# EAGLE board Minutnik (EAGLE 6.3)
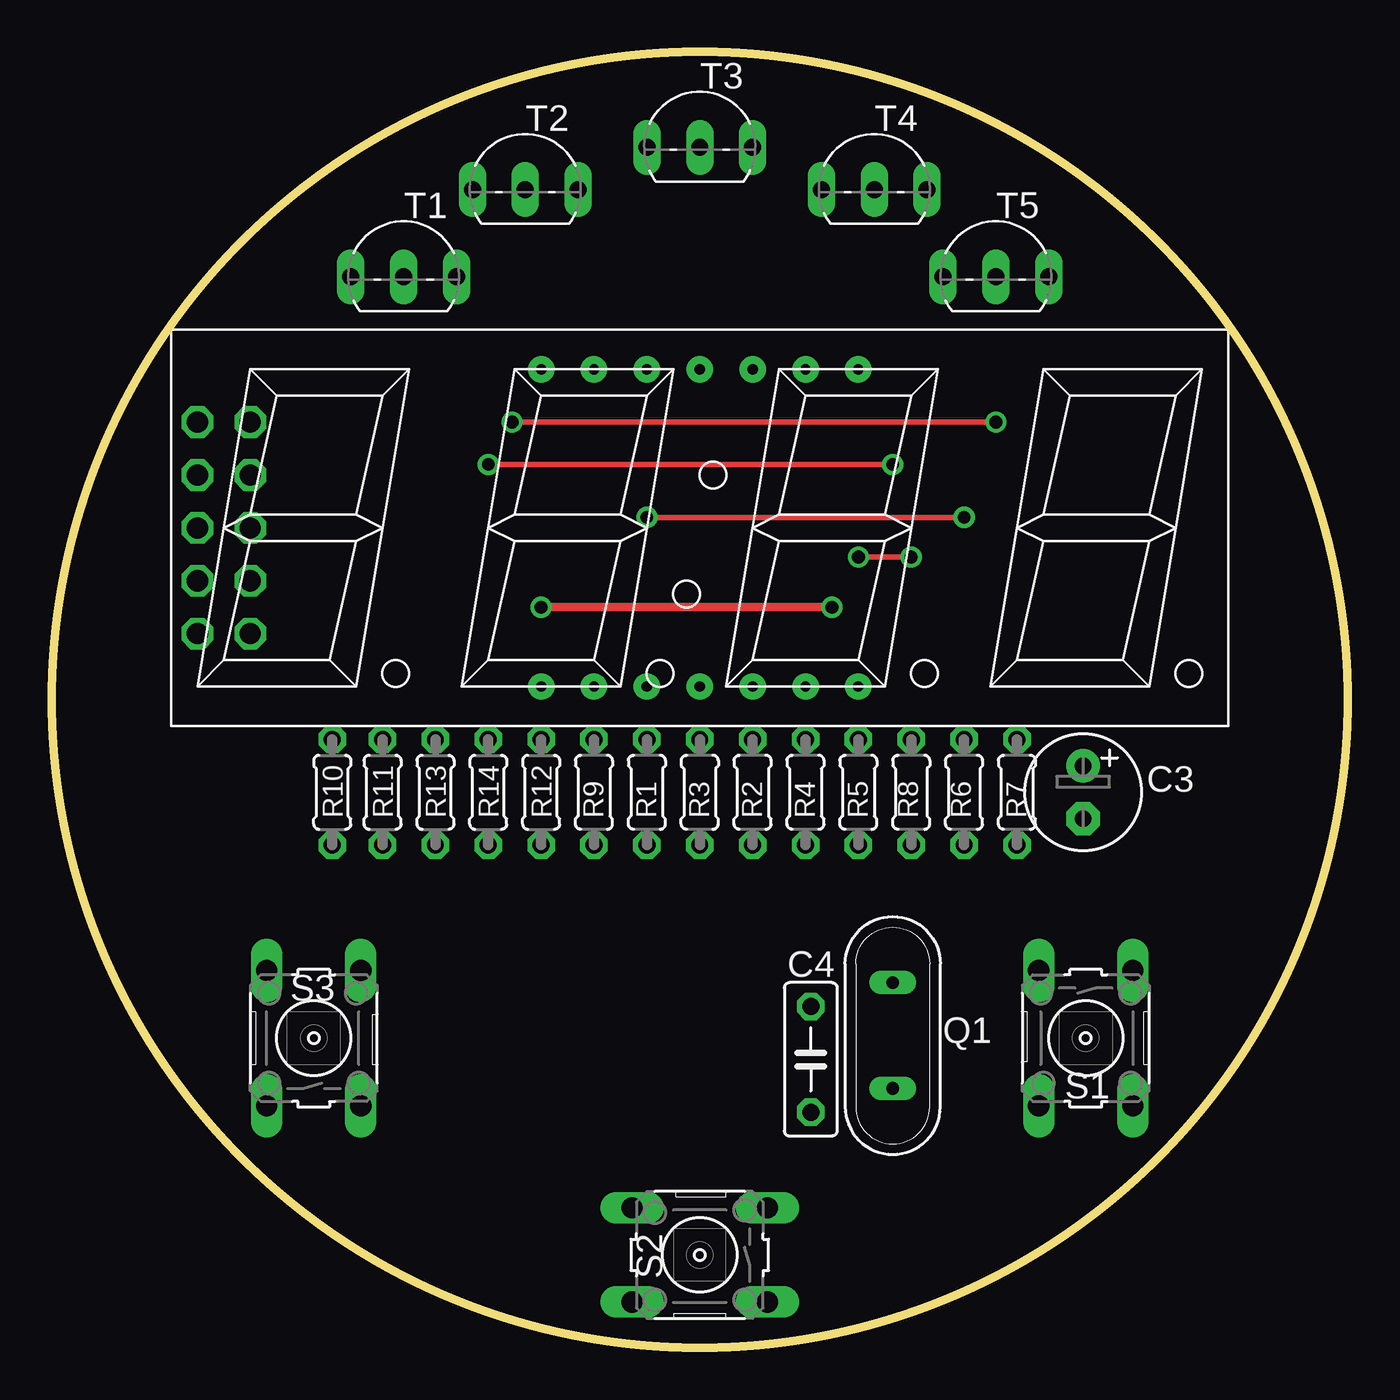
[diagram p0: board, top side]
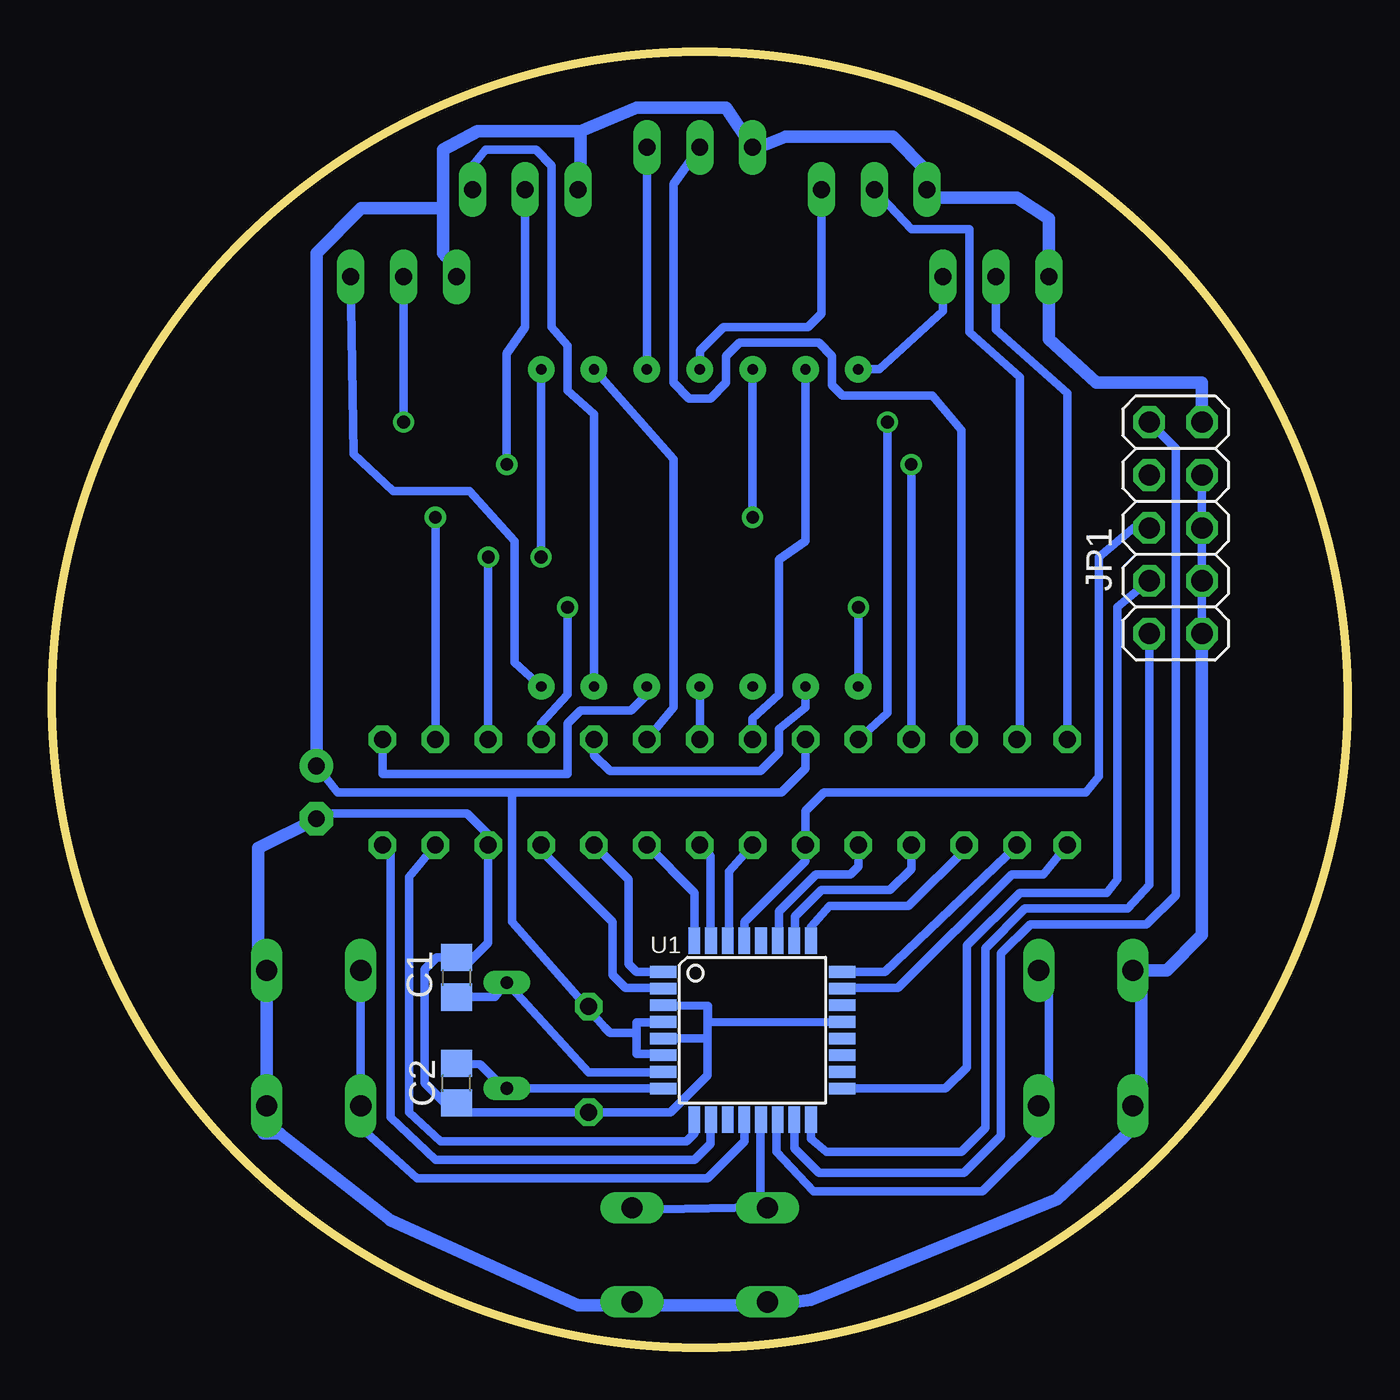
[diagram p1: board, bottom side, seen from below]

Size 62.23 x 62.23 mm. Coordinates in mm from the lower left corner, seen from the top.
Outline: circle at 31.11,31.11 radius 31.11
Copper layers (1*16): Top 0.035mm / dielectric 1.5mm / Bottom 0.035mm
Design rules "default": minimum track width 10mil, minimum drill 24mil, track to track 8mil, track to pad 8mil, pad to pad 8mil, via to via 8mil, smd to smd 8mil, copper to edge 40mil, drill to drill 8mil, minimum pad ring 10mil, minimum via ring 8mil, stop-mask expansion 4mil, vias tented up to drill 0mil, thermal gap 10mil

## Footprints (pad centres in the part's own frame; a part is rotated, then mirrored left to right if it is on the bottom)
C0805 = smd 1.3 x 1.5: 1 -0.95,0; 2 0.95,0
E2,5-6 = drill 0.813 pad 1.6: + -1.27,0 | drill 0.813 pad 1.6 octagon: - 1.27,0
C050-025X075 = drill 0.813 octagon: 1 -2.54,0; 2 2.54,0
2X05 = drill 1.016 octagon: 1 -5.08,-1.27; 2 -5.08,1.27; 3 -2.54,-1.27; 4 -2.54,1.27; 5 0,-1.27; 6 0,1.27; 7 2.54,-1.27; 8 2.54,1.27; 9 5.08,-1.27; 10 5.08,1.27
QS = drill 0.61 long: 1 -2.54,0; 2 2.54,0
0204/5 = drill 0.813 octagon: 1 -2.54,0; 2 2.54,0
B3F-10XX = drill 1.016 long: 1 -3.251,2.261; 2 3.251,2.261; 3 -3.251,-2.261; 4 3.251,-2.261
TO92-EBC = drill 0.813 long: B 0,-1.27; C -2.54,-1.27; E 2.54,-1.27
TQFP32-08 = smd 1.27 x 0.559: 1 -4.293,2.8; 2 -4.293,2; 3 -4.293,1.2; 4 -4.293,0.4; 5 -4.293,-0.4; 6 -4.293,-1.2; 7 -4.293,-2; 8 -4.293,-2.8; 17 4.293,-2.8; 18 4.293,-2; 19 4.293,-1.2; 20 4.293,-0.4; 21 4.293,0.4; 22 4.293,1.2; 23 4.293,2; 24 4.293,2.8 | smd 0.559 x 1.27: 9 -2.8,-4.293; 10 -2,-4.293; 11 -1.2,-4.293; 12 -0.4,-4.293; 13 0.4,-4.293; 14 1.2,-4.293; 15 2,-4.293; 16 2.8,-4.293; 25 2.8,4.293; 26 2,4.293; 27 1.2,4.293; 28 0.4,4.293; 29 -0.4,4.293; 30 -1.2,4.293; 31 -2,4.293; 32 -2.8,4.293
TOF-5462DX = drill 0.5 pad 1.27: A -5.08,7.62; A1 -7.62,7.62; A2 0,7.62; A3 2.54,7.62; A4 5.08,-7.62; ADOT 7.62,-7.62; B 5.08,7.62; C 0,-7.62; D -5.08,-7.62; DOT 7.62,7.62; DP -2.54,-7.62; E -7.62,-7.62; F -2.54,7.62; G 2.54,-7.62

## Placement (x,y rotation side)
C1  22pF  [C0805]  42.8,17.78 270 bottom
C2  22pF  [C0805]  42.8,12.7 90 bottom
C3  100uF  [E2,5-6]  49.53,26.67 270 top
C4  100nF  [C050-025X075]  36.45,13.84 270 top
JP1  [2X05]  8.25,39.37 270 bottom
Q1  [QS]  40.39,14.99 90 top
R1  [0204/5]  28.57,26.67 90 top
R2  [0204/5]  33.66,26.67 90 top
R3  [0204/5]  31.11,26.67 90 top
R4  [0204/5]  36.19,26.67 90 top
R5  [0204/5]  38.73,26.67 90 top
R6  [0204/5]  43.81,26.67 90 top
R7  [0204/5]  46.36,26.67 90 top
R8  [0204/5]  41.27,26.67 90 top
R9  1k  [0204/5]  26.04,26.67 90 top
R10  10k  [0204/5]  13.46,26.67 270 top
R11  10k  [0204/5]  15.88,26.67 270 top
R12  10k  [0204/5]  23.49,26.67 270 top
R13  10k  [0204/5]  18.41,26.67 270 top
R14  10k  [0204/5]  20.95,26.67 270 top
S1  [B3F-10XX]  49.66,14.86 270 top
S2  [B3F-10XX]  31.11,4.44 180 top
S3  [B3F-10XX]  12.57,14.86 90 top
T1  BC548  [TO92-EBC]  16.89,52.7 0 top
T2  BC548  [TO92-EBC]  22.73,56.9 0 top
T3  BC548  [TO92-EBC]  31.11,58.93 0 top
T4  BC548  [TO92-EBC]  39.5,56.9 0 top
T5  BC548  [TO92-EBC]  45.34,52.7 0 top
U1  ATmega8L  [TQFP32-08]  28.57,15.24 0 bottom
U$1  TOF-5462DX  [TOF-5462DX]  31.11,39.37 0 top

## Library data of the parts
C1-C4 R1-R14 = rcl
JP1 = pinhead
Q1 = special
S1-S3 = switch-omron
T1-T5 = transistor-npn
U1 = atmel
U$1 = 7seg led disp

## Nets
+5V: C3.+ C4.1 JP1.2 R9.2 T1.C T2.C T3.C T4.C T5.C U1.4 U1.6
A: R1.1 U1.30
A1: R10.2 U1.23
A2: R11.2 U1.24
A3: R13.2 U1.25
A4: R14.2 U1.26
AVCC: U1.18
B: R2.1 U1.32
BUZZ: JP1.1 U1.15
C: R3.1 U1.31
D: R4.1 U1.1
DOT: R12.2 U1.27
E: R5.1 U1.2
F: R6.1 U1.9
G: R7.1 U1.10
GND: C1.1 C2.1 C3.- C4.2 JP1.4 JP1.6 JP1.8 JP1.10 R8.1 S1.1 S1.2 S2.1 S2.2 S3.1 S3.2 U1.3 U1.5 U1.21
MISO: JP1.9 U1.16
N$1: T1.E U$1.A1
N$2: T2.E U$1.A2
N$3: T5.E U$1.ADOT
N$4: T3.E U$1.A3
N$5: T4.E U$1.A4
N$6: R1.2 U$1.A
N$7: R2.2 U$1.B
N$8: R3.2 U$1.C
N$9: R4.2 U$1.D
N$10: R5.2 U$1.E
N$11: R6.2 U$1.F
N$12: R7.2 U$1.G
N$13: R8.2 U$1.DOT
N$14: C1.2 Q1.2 U1.7
N$15: C2.2 Q1.1 U1.8
N$17: R14.1 T4.B
N$18: R13.1 T3.B
N$19: R12.1 T5.B
N$20: R11.1 T2.B
N$21: R10.1 T1.B
RST: JP1.5 R9.1 U1.29
S1: S1.3 S1.4 U1.12
S2: S2.3 S2.4 U1.13
S3: S3.3 S3.4 U1.14
SCK: JP1.7 U1.17

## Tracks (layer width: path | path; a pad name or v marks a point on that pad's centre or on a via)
+5V
  Bottom 0.254: 32.89,14.1 U1.6 | 33.4,15.62 U1.4 | C3.+ 49.53,28.19 | 36.45,16.26 C4.1
  Bottom 0.406: 42.8,51.82 T5.C | 32.89,14.1 34.16,14.1 34.16,15.11 | 34.16,15.11 34.16,15.62 33.4,15.62 | 34.16,15.11 35.43,15.11 35.69,15.37 36.45,16.26 40.13,20.45 40.13,26.67 | 40.13,26.67 48.51,26.67 C3.+ | R9.2 26.04,27.81 27.18,26.67 40.13,26.67
  Bottom 0.61: T4.C 36.83,56.13 36.83,58.42 | 36.83,58.42 41.78,58.42 43.43,57.53 43.43,54.74 | 43.43,54.74 43.43,52.58 42.8,51.82 | 36.83,58.42 34.16,59.56 29.84,59.56 T3.C 28.26,57.66 26.99,58.17 21.84,58.17 20.19,56.52 T2.C 19.81,55.25 15.88,55.25 14.35,54.23 T1.C 14.35,48.45 12.06,46.36 6.98,46.36 JP1.2 | 49.53,28.19 49.53,52.58 47.37,54.74 43.43,54.74
A
  Bottom 0.254: 29.72,19.56 U1.30
  Bottom 0.406: 29.72,19.56 29.72,22.86 R1.1
A1
  Bottom 0.254: U1.23 24.26,17.27
  Bottom 0.406: 24.26,17.27 21.59,17.27 16.13,22.73 14.6,22.73 R10.2
A2
  Bottom 0.254: U1.24 24.13,18.03
  Bottom 0.406: 24.13,18.03 22.22,18.03 16.38,23.62 R11.2
A3
  Bottom 0.406: R13.2 18.29,24.13 18.29,24 21.08,21.21 24.89,21.21 25.78,20.19 25.78,19.94 U1.25
A4
  Bottom 0.254: 26.54,19.56 U1.26
  Bottom 0.406: 26.54,19.56 26.54,20.7 25.27,21.97 21.97,21.97 20.95,22.99 R14.2
B
  Bottom 0.406: R2.1 31.37,21.84 U1.32
BUZZ
  Bottom 0.406: JP1.1 8.25,43.18 8.25,21.72 9.65,20.32 15.24,20.32 16.64,18.92 16.64,10.16 18.41,8.38 25.4,8.38 26.57,9.56 U1.15
C
  Bottom 0.406: R3.1 30.61,23.62 30.61,19.56 U1.31
D
  Bottom 0.406: R4.1 34.54,22.48 34.54,18.41 34.16,18.03 33.78,18.03 U1.1
DOT
  Bottom 0.254: 27.3,19.56 U1.27
  Bottom 0.406: 27.3,19.56 27.3,20.95 25.53,22.73 23.88,22.73 23.49,23.11 R12.2
E
  Bottom 0.254: 32.89,17.27 U1.2
  Bottom 0.406: 32.89,17.27 34.67,17.27 35.31,17.91 35.31,20.45 38.61,23.75 R5.1
F
  Bottom 0.406: R6.1 45.08,22.61 45.08,11.3 43.56,9.91 31.75,9.91 31.37,10.29 U1.9
G
  Bottom 0.406: R7.1 45.97,23.75 45.97,11.05 43.81,9.02 31.37,9.02 30.61,9.78 30.61,10.92 U1.10
GND
  Bottom 0.254: 34.29,2.03 S2.1 34.42,2.03 | 32.89,14.86 U1.5 | 32.89,16.38 U1.3 32.77,16.38 | U1.21 24.26,15.62 | 28.07,2.03 S2.2 | 6.98,34.8 JP1.10 | 52.32,17.27 S1.1
  Bottom 0.406: 9.91,10.79 S3.1 10.03,10.79 | 6.98,34.8 JP1.8 JP1.6 JP1.4 | U1.21 30.73,15.62 30.73,16.38 30.73,16.42 | 30.73,16.42 U1.3 | 30.73,14.86 32.89,14.86 | 30.73,14.86 30.73,16.42 | 30.73,14.86 30.73,13.08 32.51,11.3 C4.2 42.8,11.3 C2.1 43.37,11.75 44.32,12.7 44.32,18.16 43.75,18.73 C1.1 43.05,18.41 | 43.05,18.41 42.29,18.41 41.27,19.43 R8.1 41.27,24.64 42.29,25.65 49.91,25.65 C3.- | 43.05,18.41 43.05,19.05
  Bottom 0.61: 34.29,2.03 28.07,2.03 27.69,2.03 25.78,2.29 13.97,7.11 10.03,10.79 | S1.1 S1.2 52.07,10.29 51.31,10.29 45.97,6.1 36.96,2.03 34.42,2.03 | 9.91,10.79 9.91,17.14 S3.2 8.69,18.11 6.98,19.81 6.98,34.8 | C3.- 52.32,24 52.32,17.27
MISO
  Bottom 0.406: JP1.9 9.52,22.22 10.54,21.08 15.49,21.08 17.4,19.18 17.4,10.54 18.54,9.4 25.02,9.4 25.78,10.03 U1.16
N$1
  Bottom 0.406: U$1.A1 22.48,46.99 19.43,49.78 T1.E
N$2
  Bottom 0.406: T2.E 25.27,49.66 25.91,49.02 29.97,49.02 31.11,47.88 U$1.A2
N$3
  Bottom 0.406: U$1.ADOT 40,32.89 40,38.73 42.16,41.15 45.85,41.15 47.75,42.93 T5.E
N$4
  Bottom 0.406: U$1.A3 T3.E
N$5
  Bottom 0.254: 42.04,56.77 T4.E
  Bottom 0.406: U$1.A4 36.19,44.83 37.47,45.97 37.47,48.13 38.23,49.02 38.23,56.77 38.99,57.53 41.4,57.53 42.04,56.77
N$6
  Bottom 0.406: U$1.A 26.04,38.73 27.3,37.85 27.3,31.37 28.57,30.23 R1.2
N$7
  Bottom 0.406: U$1.B 32.39,42.67 32.39,30.73 R2.2
N$8
  Bottom 0.406: U$1.C R3.2
N$9
  Bottom 0.406: U$1.D 26.04,30.73 27.3,29.72 27.3,28.57 28.19,27.69 35.43,27.69 36.19,28.45 R4.2
N$10  (via drill 0.61)
  Top 0.406: v23.49,35.56 v37.47,35.56
  Bottom 0.406: v23.49,35.56 U$1.E | v37.47,35.56 37.47,31.37 38.73,29.97 R5.2
N$11  (via drill 0.61)
  Top 0.254: v28.57,39.88 v43.81,39.88
  Bottom 0.406: v28.57,39.88 U$1.F | v43.81,39.88 R6.2
N$12
  Bottom 0.406: R7.2 46.36,27.56 37.47,27.56 37.47,29.97 36.83,30.61 34.42,30.61 33.66,31.37 U$1.G
N$13  (via drill 0.61)
  Top 0.254: v41.27,37.97 v38.73,37.97
  Bottom 0.406: v38.73,37.97 U$1.DOT | R8.2 v41.27,37.97
N$14
  Bottom 0.254: 32.89,13.21 U1.7
  Bottom 0.406: 32.89,13.21 36.45,13.21 Q1.2 40.95,16.83 C1.2
N$15
  Bottom 0.254: 33.4,12.45 U1.8
  Bottom 0.406: 33.4,12.45 Q1.1 40.51,12.45 41.66,13.59 C2.2
N$17  (via drill 0.61)
  Top 0.254: v20.95,42.42 v40.39,42.42
  Bottom 0.406: v20.95,42.42 R14.1 | v40.39,42.42 40.39,47.75 39.5,49.02 T4.B
N$18
  Bottom 0.254: 18.54,29.97 R13.1
  Bottom 0.406: T3.B 32.39,55.88 32.39,46.36 31.62,45.59 30.61,45.59 29.84,46.36 29.84,47.62 29.21,48.26 25.4,48.26 24.76,47.62 24.76,46.23 24.26,45.72 19.94,45.72 18.54,44.07 18.54,29.97
N$19  (via drill 0.61)
  Top 0.254: v22.1,44.45 v45.34,44.45
  Bottom 0.406: R12.1 22.1,30.48 v22.1,44.45 | v45.34,44.45 T5.B
N$20
  Bottom 0.406: R11.1 15.75,29.21 15.75,46.61 18.16,48.77 18.16,53.72 20.95,53.72 T2.B
N$21
  Bottom 0.406: R10.1 13.46,45.85 16.89,48.89 T1.B
RST
  Bottom 0.254: 28.96,19.68 28.96,19.56 U1.29
  Bottom 0.406: 28.96,19.68 28.96,20.45 26.04,23.37 R9.1 26.04,25.78 25.15,26.67 12.57,26.67 11.94,27.43 11.94,37.97 10.29,39.37 JP1.5
S1
  Bottom 0.254: 28.96,10.79 U1.12 | S1.4 47.37,10.54
  Bottom 0.406: S1.4 S1.3 | 28.96,10.79 28.96,9.91 30.73,8.13 44.7,8.13 47.37,10.54
S2
  Bottom 0.254: 28.19,6.73 27.94,6.6 S2.4 | 28.19,10.79 U1.13 | S2.3 34.29,6.6
  Bottom 0.406: 28.19,6.73 28.19,10.79 | 34.29,6.6 28.19,6.73 | 28.19,6.73 S2.4
S3
  Bottom 0.254: U1.14 27.43,10.92 | 14.35,10.67 S3.3 14.35,10.79 | 14.35,17.14 S3.4
  Bottom 0.406: 27.43,10.92 27.43,9.4 25.65,7.49 17.53,7.49 14.35,10.67 | 14.35,10.79 14.35,17.14
SCK
  Bottom 0.254: 24.26,12.45 U1.17
  Bottom 0.406: 24.26,12.45 19.3,12.45 18.29,13.46 18.29,19.3 15.75,21.84 11.56,21.84 11.05,22.48 11.05,35.56 JP1.7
